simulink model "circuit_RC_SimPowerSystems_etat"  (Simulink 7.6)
settings: Solver=ode15s  StartTime=0.0  StopTime=0.04  RelTol=1e-3
InitFcn:
  | R=2;
  | C=1e-3;
StopFcn:
  | load Vc_I_Creneau.mat
  | plot(x(1,:),x(2,:),x(1,:),x(3,:),x(1,:),x(4,:))
  | axis([0 0.04 -60 120])
  | grid
  | title('tension Vc, courant I et créneau d''entrée')
  | xlabel('temps')
libraries: powerlib x8

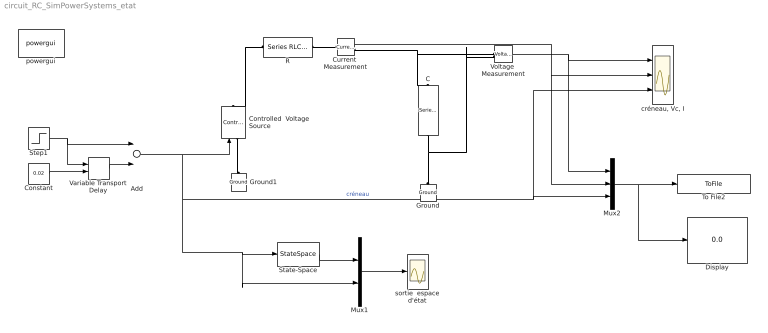
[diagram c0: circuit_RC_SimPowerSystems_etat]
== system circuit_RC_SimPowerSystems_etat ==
  Add : Sum  Inputs=+-
  C : powerlib/Elements/Series RLC Branch  DialogController=POWERSYS.PowerSysDialog  PhysicalDomain=powersysdomain  SubClassName=unknown  LeftPortType=p1  RightPortType=p1  LConnTagsString=__new0  RConnTagsString=__new0  BranchType=C  Resistance=R  Inductance=1e-3  SetiL0=off  InitialCurrent=0  Capacitance=C  Setx0=off  InitialVoltage=0  Measurements=None
  Constant : Constant  Value=0.02
  Controlled  Voltage Source : powerlib/Electrical Sources/Controlled Voltage Source  DialogController=POWERSYS.PowerSysDialog  SystemSampleTime=-1  Initialize=on  Source_Type=AC  Amplitude=0  Phase=0  Frequency=0  Measurements=None
  Current  Measurement : powerlib/Measurements/Current Measurement  DialogController=POWERSYS.PowerSysDialog  SystemSampleTime=-1  PhasorSimulation=off  OutputType=Complex  PSBequivalent=0
  Display : Display
  Ground : powerlib/Elements/Ground  DialogController=POWERSYS.PowerSysDialog  PhysicalDomain=powersysdomain  SubClassName=unknown  LeftPortType=p1  RightPortType=p1  LConnTagsString=a
  Ground1 : powerlib/Elements/Ground  DialogController=POWERSYS.PowerSysDialog  PhysicalDomain=powersysdomain  SubClassName=unknown  LeftPortType=p1  RightPortType=p1  LConnTagsString=a
  Mux1 : Mux  Inputs=2
  Mux2 : Mux  Inputs=3
  R : powerlib/Elements/Series RLC Branch  DialogController=POWERSYS.PowerSysDialog  PhysicalDomain=powersysdomain  SubClassName=unknown  LeftPortType=p1  RightPortType=p1  LConnTagsString=__new0  RConnTagsString=__new0  BranchType=R  Resistance=R  Inductance=1e-3  SetiL0=off  InitialCurrent=0  Capacitance=1e-6  Setx0=off  InitialVoltage=0  Measurements=None
  State-Space : StateSpace  A=-1/(R*C)  B=1/(R*C)  C=[1 -1/R]'  D=[0 1/R]'
  Step1 : Step  Time=0.005  After=100  SampleTime=0
  To File2 : ToFile  Filename=Vc_I_Creneau  MatrixName=x
  Variable Transport Delay : VariableTransportDelay  VariableDelayType=Variable transport delay  MaximumDelay=10
  Voltage  Measurement : powerlib/Measurements/Voltage Measurement  DialogController=POWERSYS.PowerSysDialog  SystemSampleTime=-1  PhasorSimulation=off  OutputType=Complex  PSBequivalent=0
  "créneau, Vc, I" : Scope  NumInputPorts=3
  powergui : powerlib/powergui  Priority=1  SystemSampleTime=-1  SimulationMode=Continuous  SampleTime=50e-6  frequency=60  SPID=off  DisableSnubberDevices=off  DisableRonSwitches=off  DisableVfSwitches=off  SwTol=0  Interpol=off  frequencyindice=0  echomessages=off  HookPort=off  DisplayEquations=off  FunctionMessages=off  EnableUseOfTLC=off  x0status=blocks  RestoreLinks=warning  ResistiveCurrentMeasurement=off  Ylog=off  Xlog=on  ShowGrid=off  save=off  variable=ZData  ZoomFFT=off  StartTime=0.0  cycles=1  DisplayStyle=1  FreqAxis=off  MaxFrequency=1000  frequencyindicesteady=1  display=off  methode=off
  sortie  espace d'état : Scope
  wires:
  Add/1 -> Controlled  Voltage Source/1, "créneau, Vc, I"/3, Mux2/3, State-Space/1, Mux1/2  "créneau"
  Step1/1 -> Variable Transport Delay/1, Add/1
  Variable Transport Delay/1 -> Add/2
  Constant/1 -> Variable Transport Delay/2
  Voltage  Measurement/1 -> "créneau, Vc, I"/1, Mux2/1
  Current  Measurement/1 -> "créneau, Vc, I"/2, Mux2/2
  Mux2/1 -> To File2/1, Display/1
  State-Space/1 -> Mux1/1
  Mux1/1 -> sortie  espace d'état/1
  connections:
  C/RConn1 -- Ground/LConn1 -- Voltage  Measurement/LConn2
  R/LConn1 -- Controlled  Voltage Source/RConn1
  R/RConn1 -- Current  Measurement/LConn1
  Current  Measurement/RConn1 -- C/LConn1 -- Voltage  Measurement/LConn1
  Controlled  Voltage Source/LConn1 -- Ground1/LConn1
